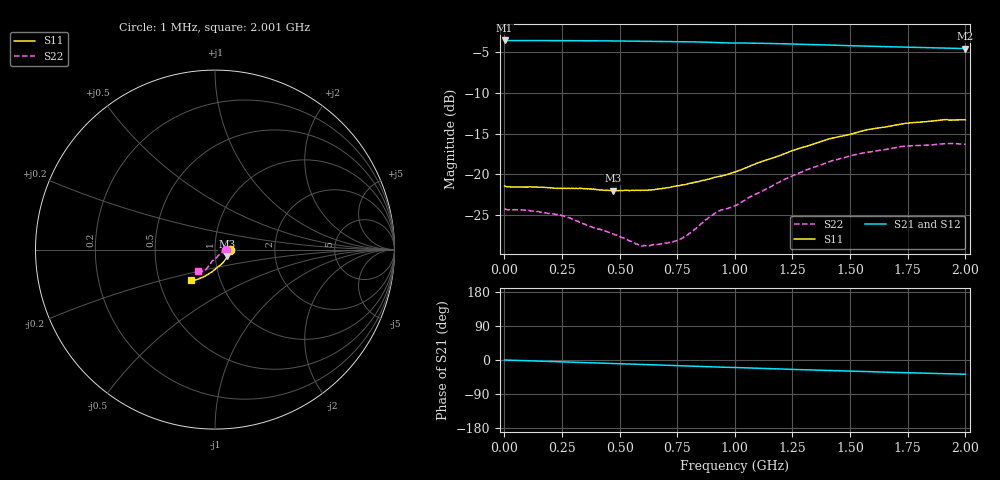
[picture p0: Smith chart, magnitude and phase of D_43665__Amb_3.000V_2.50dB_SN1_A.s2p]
! device id: 43665_
! dir: \\malibu\benchdata\1_engineers\tn_data\43665_75ohm\new\sparar\43665_\amb\3p000v\2p50db
! Serial: 1
! Insertion: A
! Temp: Amb
! VDD: 3.000V
! Attenuation Step: 2.50dB
! IDD: 1.450573e+00mA
! FILE NAME
! DATE 03-27-2009 08:33:59
! CORRECTED  DATA
#  Hz  S  RI  R  75
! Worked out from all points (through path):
!   401 points, 1 MHz to 2.001 GHz, reference 75 ohm
!   highest |S21| = -3.56 dB at 1 MHz (marker M1); lowest = -4.6 dB at 2.001 GHz (marker M2)
!   group delay of S21, straight-line fit = 53.2 ps
!   lowest |S11| = -22.0 dB at 471 MHz (marker M3), VSWR 1.17, Z = 85.9 - j6.6 ohm
!   |S11| at or under -10 dB: start of sweep to end of sweep
!   |S22| runs from -28.8 to -16.2 dB; largest |S21 - S12| = 0.0036
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1000000  0.085 -0.00139  0.6639 -0.00105  0.6643 -0.00111  0.0616 -0.000954
9.6e7  0.0833 -0.00658  0.6625 -0.0215  0.6627 -0.0214  0.0604 -0.00105
2.36e8  0.0805 -0.0171  0.66 -0.0527  0.6603 -0.0526  0.0563 -0.00415
3.36e8  0.0779 -0.0259  0.6568 -0.0753  0.6571 -0.0749  0.05 -0.00637
4.71e8  0.0695 -0.0381  0.6509 -0.1055  0.6513 -0.1051  0.041 -0.0139
5.91e8  0.0605 -0.0518  0.6433 -0.1321  0.6436 -0.1316  0.0297 -0.0217
6.21e8  0.0577 -0.0553  0.6414 -0.1386  0.6417 -0.1381  0.027 -0.0242
6.71e8  0.0529 -0.0619  0.6381 -0.1499  0.6384 -0.1492  0.0232 -0.0292
7.61e8  0.0434 -0.0736  0.6304 -0.1701  0.6309 -0.1692  0.0143 -0.0374
8.01e8  0.0384 -0.0791  0.6265 -0.1791  0.6271 -0.1782  0.00944 -0.0422
8.76e8  0.027 -0.0888  0.6178 -0.1958  0.6185 -0.1948  0.00186 -0.0529
9.21e8  0.0193 -0.0944  0.6109 -0.2047  0.6118 -0.2035  -0.00456 -0.0583
1.001e9  0.00919 -0.103  0.603 -0.2167  0.6042 -0.2157  -0.0158 -0.0621
1.211e9  -0.0275 -0.1304  0.5788 -0.2577  0.5805 -0.2573  -0.0313 -0.0871
1.336e9  -0.0502 -0.1441  0.5611 -0.2782  0.5631 -0.2778  -0.0432 -0.1007
1.406e9  -0.0634 -0.1519  0.5509 -0.2901  0.5528 -0.2904  -0.048 -0.1091
1.511e9  -0.0809 -0.1583  0.5357 -0.3041  0.5374 -0.3047  -0.06 -0.1165
1.576e9  -0.0914 -0.1642  0.5267 -0.3132  0.5282 -0.3144  -0.0642 -0.1209
1.671e9  -0.1048 -0.1675  0.5132 -0.3251  0.5139 -0.326  -0.0735 -0.1235
1.746e9  -0.1145 -0.1714  0.5026 -0.334  0.5033 -0.3352  -0.0795 -0.1264
1.911e9  -0.1302 -0.1732  0.4805 -0.3517  0.4807 -0.3514  -0.0931 -0.1231
2.001e9  -0.1325 -0.171  0.4701 -0.3599  0.468 -0.3615  -0.0974 -0.1182
